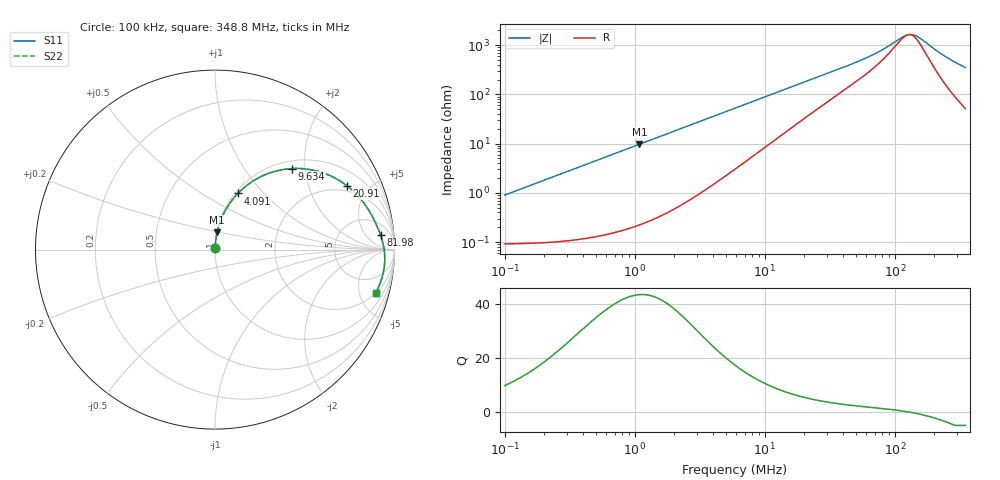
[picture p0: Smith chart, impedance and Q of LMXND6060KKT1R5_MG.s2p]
! LMXND6060KKT1R5_MG  S-PARAMETER MODEL  ( General Type )
! Model Generated by TAIYO YUDEN Corporation (http://www.ty-top.com)
! Version 1.0
! TAIYO YUDEN Control No. 191023NI43SB-FBB
! Copyright(c) 2019 TAIYO YUDEN CO.,LTD. All Rights Reserved.
! Product Description (link to TY-COMPAS)
! https://ds.yuden.co.jp/TYCOMPAS/or/detail?pn=LMXND6060KKT1R5MMG&u=M
! Products Name : Inductors
! Characteristics :
!  Inductance : 1.5 uH , SRF(min) : 77 MHz , DC Resistance(max) : 0.108 Ohm
!  Rated Current : Saturation :2400 mA , Temp Rise : 1900 mA
!  Case Size : 6.0 x 6.0 / 0.236 x 0.236 [mm/inch] , Thickness : 1 / 0.039 [mm/inch]
!  (Conditions: Temperature = 25 degC , DC Bias Current/Voltage = 0A / 0V)
! External Node Assignments :
!  1  o---GGG---o  2
! GND o---------o GND
! Frequency Range : 0.1MHz  -  348.750116MHz  [ 402 STEP ]
# MHz S RI R 50
! Freq[MHz].  S11 Real  S11 Imag  S21 Real  S21 Imag  S12 Real  S12 Imag  S22 Real  S22 Imag
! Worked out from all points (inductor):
!   401 points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, 100 kHz to 348.8 MHz, reference 50 ohm
!   read as one part in series: L = 1.43 uH near 104.2 kHz
!   highest Q = 43.5 at 1.087 MHz (marker M1), where L = 1.42 uH
!   self-resonance near 127.2 MHz
!   S11 on the Smith chart (normalised r, x): 100 kHz: 1.00, +0.02; 4.091 MHz: 1.03, +0.73; 9.634 MHz: 1.16, +1.71; 20.91 MHz: 1.70, +3.63; 81.98 MHz: 12, +13; 348.8 MHz: 2.03, -6.95
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0.1  0.000999 0.00897  0.999 -0.00897  0.999 -0.00897  0.000999 0.00897
0.392077  0.00238 0.035  0.9976 -0.035  0.9976 -0.035  0.00238 0.035
1.08689  0.0115 0.0957  0.9885 -0.0957  0.9885 -0.0957  0.0115 0.0957
1.537242  0.0215 0.1338  0.9785 -0.1338  0.9785 -0.1338  0.0215 0.1338
2.666012  0.0595 0.2218  0.9405 -0.2218  0.9405 -0.2218  0.0595 0.2218
4.091137  0.1274 0.3131  0.8726 -0.3131  0.8726 -0.3131  0.1274 0.3131
5.905507  0.2295 0.3927  0.7705 -0.3927  0.7705 -0.3927  0.2295 0.3927
9.634031  0.4297 0.4516  0.5703 -0.4516  0.5703 -0.4516  0.4297 0.4516
13.62589  0.5837 0.4334  0.4163 -0.4334  0.4163 -0.4334  0.5837 0.4334
20.90966  0.7365 0.3548  0.2635 -0.3548  0.2635 -0.3548  0.7365 0.3548
23.15412  0.764 0.3318  0.236 -0.3318  0.236 -0.3318  0.764 0.3318
32.74803  0.8345 0.2528  0.1655 -0.2528  0.1655 -0.2528  0.8345 0.2528
50.2536  0.8866 0.1657  0.1134 -0.1657  0.1134 -0.1657  0.8866 0.1657
65.50869  0.9082 0.1181  0.0918 -0.1181  0.0918 -0.1181  0.9082 0.1181
81.98192  0.9228 0.0795  0.0772 -0.0795  0.0772 -0.0795  0.9228 0.0795
90.78195  0.9285 0.0618  0.0715 -0.0618  0.0715 -0.0618  0.9285 0.0618
120.7779  0.9409 0.0099  0.0591 -0.0099  0.0591 -0.0099  0.9409 0.0099
131.0426  0.9432 -0.00585  0.0568 0.00585  0.0568 0.00585  0.9432 -0.00585
139.3097  0.9445 -0.018  0.0555 0.018  0.0555 0.018  0.9445 -0.018
157.4415  0.9459 -0.0432  0.0541 0.0432  0.0541 0.0432  0.9459 -0.0432
246.5798  0.9328 -0.1479  0.0672 0.1479  0.0672 0.1479  0.9328 -0.1479
348.7501  0.8946 -0.2418  0.1054 0.2418  0.1054 0.2418  0.8946 -0.2418
